| TEXAS INSTRUMENTS INCORPORATED
| Standard Linear and Logic Group
| IBIS Model of TS3DV416
| 4-CHANNEL DIFFERENTIAL 8:16 MULTIPLEXER SWITCH FOR DVI/HDMI
| APLICATIONS
| This file contains package information for the following:
|  TSSOP 48-pin (DGG) package as [Component] TS3DV416DB_DGG
|  TVSOP 48-pin (DGV) package as [Component] TS3DV416DB_DGV
| This device can be powered at the following Vccs:
|  3.3 volt Vcc
| This file provides unique models under the [Model Selector] for each Vcc.
| For operation at a specific Vcc, select the appropriate model after each
| [Model Selector] keyword.
[IBIS Ver]   3.2
[Comment char]  |_char
[File Name]   ts3dv416.ibs
[File Rev]   1.1 | b_die
[Date]   September 22, 2006
[Source]   Data created from TI-SPICE simulations at TI-SLL.
[Notes]   The following is an IBIS list for the TS3DV416.
   Please contact sllibis@ti.com with questions and
   comments concerning SLL IBIS models.
   - FILE REV HISTORY
   - 1.1 Release IBIS file on 09/22/06
   - Power clamp data deleted as there is no power-clamp diode.
[Disclaimer] Property of Texas Instruments Incorporated.  Unauthorized
   reproduction and/or distribution is strictly prohibited.
   This product is protected under copyright law.
   Created  2005, (C) Copyright  2005, Texas Instruments
   Incorporated, All Rights Reserved
   UNLESS THERE IS A SIGNED, WRITTEN AGREEMENT TO THE
   CONTRARY, TEXAS INSTRUMENTS (TI) IS PROVIDING THE IBIS
   MODELS  AND WITHOUT ANY WARRANTY, EXPRESSED OR
   IMPLIED.  TI assumes no liability for:
   1) the accuracy of the IBIS models provided to your
   company;
   2) the proper functioning of these IBIS Models in your
   design or for any resulting applications; or
   3) infringement of patents, copyrights or intellectual
   property rights resulting from your use of these IBIS
   models.
   TI provides IBIS Models as a service to our customers.
   You and your company shall not distribute, sell or give
   these models to anyone else without prior written
   permission from TI.
   TI reserves the right to make changes to our products or
   to discontinue any semiconductor product or service
   without notice, and advises our customers to obtain the
   latest version of relevant information to verify, before
   placing orders, that the information being relied on is
   current.
   Please be aware that your receipt and use of the IBIS
   information provided shall serve as acceptance of these
   terms and conditions.  If you do not accept these terms,
   you should return or destroy the IBIS models and any
   other accompanying information immediately.
| Component TS3DV416DB_DGG 48-pin TSSOP
[Component]   TS3DV416DB_DGG
[Manufacturer]   Texas Instruments, Inc.
[Package]
|   typ   min   max
R_pkg   6.200e-02   5.000e-02   7.800e-02
L_pkg   3.527e-09   3.128e-09   4.255e-09
C_pkg   5.300e-13   4.170e-13   6.850e-13
[Pin]   signal_name   model_name   R_pin   L_pin   C_pin
1   VDD   POWER   5.000e-02   4.250e-09   6.710e-13
2   A0   TS3DV416DB_A   5.700e-02   3.956e-09   6.740e-13
3   GND   GND   7.100e-02   3.922e-09   6.190e-13
4   A1   TS3DV416DB_A   7.800e-02   3.841e-09   6.180e-13
5   GND   GND   5.600e-02   3.535e-09   5.550e-13
6   VDD   POWER   5.800e-02   3.464e-09   5.030e-13
7   GND   GND   6.000e-02   3.362e-09   4.980e-13
8   A2   TS3DV416DB_A   6.100e-02   3.293e-09   4.620e-13
9   GND   GND   6.300e-02   3.240e-09   4.550e-13
10   A3   TS3DV416DB_A   6.300e-02   3.175e-09   4.420e-13
11   GND   GND   6.400e-02   3.153e-09   4.290e-13
12   VDD   POWER   6.500e-02   3.128e-09   4.180e-13
13   GND   GND   6.500e-02   3.128e-09   4.180e-13
14   NC   NC   6.400e-02   3.154e-09   4.290e-13
15   A4   TS3DV416DB_A   6.300e-02   3.174e-09   4.420e-13
16   GND   GND   6.300e-02   3.241e-09   4.550e-13
17   A5   TS3DV416DB_A   6.100e-02   3.293e-09   4.620e-13
18   GND   GND   6.000e-02   3.362e-09   4.970e-13
19   VDD   POWER   5.800e-02   3.464e-09   5.030e-13
20   GND   GND   5.600e-02   3.537e-09   5.600e-13
21   A6   TS3DV416DB_A   7.700e-02   3.839e-09   6.260e-13
22   GND   GND   7.100e-02   3.917e-09   6.270e-13
23   A7   TS3DV416DB_A   5.800e-02   3.955e-09   6.850e-13
24   SEL   TS3DV416DB_SEL   5.200e-02   4.255e-09   6.790e-13
25   7B2   TS3DV416DB_B2   5.100e-02   4.254e-09   6.760e-13
26   6B2   TS3DV416DB_B2   5.800e-02   3.957e-09   6.790e-13
27   GND   GND   7.100e-02   3.920e-09   6.210e-13
28   7B1   TS3DV416DB_B1   7.800e-02   3.843e-09   6.220e-13
29   6B1   TS3DV416DB_B1   5.600e-02   3.539e-09   5.600e-13
30   GND   GND   5.800e-02   3.466e-09   5.030e-13
31   5B2   TS3DV416DB_B2   6.000e-02   3.363e-09   4.970e-13
32   4B2   TS3DV416DB_B2   6.100e-02   3.294e-09   4.620e-13
33   GND   GND   6.300e-02   3.241e-09   4.540e-13
34   5B1   TS3DV416DB_B1   6.300e-02   3.175e-09   4.410e-13
35   4B1   TS3DV416DB_B1   6.400e-02   3.153e-09   4.290e-13
36   VDD   POWER   6.500e-02   3.129e-09   4.170e-13
37   GND   GND   6.500e-02   3.129e-09   4.170e-13
38   3B2   TS3DV416DB_B2   6.400e-02   3.152e-09   4.290e-13
39   2B2   TS3DV416DB_B2   6.400e-02   3.176e-09   4.410e-13
40   GND   GND   6.300e-02   3.241e-09   4.540e-13
41   3B1   TS3DV416DB_B1   6.100e-02   3.293e-09   4.620e-13
42   2B1   TS3DV416DB_B1   6.000e-02   3.363e-09   4.970e-13
43   GND   GND   5.800e-02   3.464e-09   5.030e-13
44   1B2   TS3DV416DB_B2   5.600e-02   3.534e-09   5.610e-13
45   0B2   TS3DV416DB_B2   7.800e-02   3.841e-09   6.260e-13
46   GND   GND   7.100e-02   3.920e-09   6.220e-13
47   1B1   TS3DV416DB_B1   5.700e-02   3.955e-09   6.770e-13
48   0B1   TS3DV416DB_B1   5.100e-02   4.252e-09   6.720e-13
| Component TS3DV416DB_DGV 48-pin TVSOP
[Component]   TS3DV416DB_DGV
[Manufacturer]   Texas Instruments, Inc.
[Package]
|   typ   min   max
R_pkg   7.000e-02   4.900e-02   8.500e-02
L_pkg   3.013e-09   2.743e-09   3.408e-09
C_pkg   3.710e-13   2.940e-13   5.110e-13
[Pin]   signal_name   model_name   R_pin   L_pin   C_pin
1   VDD   POWER   4.900e-02   3.393e-09   4.970e-13
2   A0   TS3DV416DB_A   6.000e-02   3.250e-09   5.020e-13
3   GND   GND   7.700e-02   3.310e-09   4.510e-13
4   A1   TS3DV416DB_A   8.500e-02   3.299e-09   4.040e-13
5   GND   GND   8.300e-02   3.136e-09   3.600e-13
6   VDD   POWER   7.700e-02   3.019e-09   3.630e-13
7   GND   GND   6.500e-02   2.882e-09   3.490e-13
8   A2   TS3DV416DB_A   6.600e-02   2.829e-09   3.140e-13
9   GND   GND   6.700e-02   2.796e-09   3.140e-13
10   A3   TS3DV416DB_A   6.900e-02   2.754e-09   3.080e-13
11   GND   GND   7.000e-02   2.753e-09   3.010e-13
12   VDD   POWER   7.100e-02   2.745e-09   2.940e-13
13   GND   GND   7.000e-02   2.744e-09   2.940e-13
14   NC   NC   7.000e-02   2.754e-09   3.010e-13
15   A4   TS3DV416DB_A   6.900e-02   2.754e-09   3.080e-13
16   GND   GND   6.700e-02   2.796e-09   3.140e-13
17   A5   TS3DV416DB_A   6.600e-02   2.829e-09   3.140e-13
18   GND   GND   6.500e-02   2.883e-09   3.500e-13
19   VDD   POWER   7.500e-02   3.014e-09   3.630e-13
20   GND   GND   8.000e-02   3.128e-09   3.580e-13
21   A6   TS3DV416DB_A   8.400e-02   3.295e-09   4.030e-13
22   GND   GND   7.800e-02   3.311e-09   4.520e-13
23   A7   TS3DV416DB_A   6.200e-02   3.259e-09   5.010e-13
24   SEL   TS3DV416DB_SEL   5.200e-02   3.404e-09   4.960e-13
25   7B2   TS3DV416DB_B2   5.300e-02   3.397e-09   5.050e-13
26   6B2   TS3DV416DB_B2   6.200e-02   3.249e-09   5.110e-13
27   GND   GND   7.700e-02   3.308e-09   4.530e-13
28   7B1   TS3DV416DB_B1   8.200e-02   3.289e-09   4.030e-13
29   6B1   TS3DV416DB_B1   7.800e-02   3.121e-09   3.590e-13
30   GND   GND   7.400e-02   3.010e-09   3.630e-13
31   5B2   TS3DV416DB_B2   6.500e-02   2.883e-09   3.490e-13
32   4B2   TS3DV416DB_B2   6.700e-02   2.829e-09   3.140e-13
33   GND   GND   6.700e-02   2.795e-09   3.140e-13
34   5B1   TS3DV416DB_B1   6.900e-02   2.753e-09   3.070e-13
35   4B1   TS3DV416DB_B1   7.000e-02   2.753e-09   3.010e-13
36   VDD   POWER   7.000e-02   2.743e-09   2.940e-13
37   GND   GND   7.000e-02   2.743e-09   2.940e-13
38   3B2   TS3DV416DB_B2   7.000e-02   2.753e-09   3.010e-13
39   2B2   TS3DV416DB_B2   6.900e-02   2.754e-09   3.070e-13
40   GND   GND   6.800e-02   2.797e-09   3.140e-13
41   3B1   TS3DV416DB_B1   6.700e-02   2.830e-09   3.140e-13
42   2B1   TS3DV416DB_B1   6.400e-02   2.880e-09   3.490e-13
43   GND   GND   7.200e-02   3.004e-09   3.620e-13
44   1B2   TS3DV416DB_B2   7.800e-02   3.121e-09   3.590e-13
45   0B2   TS3DV416DB_B2   8.400e-02   3.296e-09   4.030e-13
46   GND   GND   7.700e-02   3.308e-09   4.510e-13
47   1B1   TS3DV416DB_B1   6.200e-02   3.258e-09   4.990e-13
48   0B1   TS3DV416DB_B1   5.300e-02   3.408e-09   4.940e-13
[Series Switch Groups]
| Function Group States
On  1 /   | A1-A8->1B1-8B1 SEL LOW
   | 1B1-8B1->A1-A8 SEL LOW
On  2 /   | A1-A8->1B2-8B2 SEL HIGH
   | 1B2-8B2->A1-A8 SEL HIGH
[Series Pin Mapping]   pin_2   model_name   function_table_group
2   48   TS3DV416DB_A_S   1
4   47   TS3DV416DB_A_S   1
8   42   TS3DV416DB_A_S   1
10   41   TS3DV416DB_A_S   1
15   35   TS3DV416DB_A_S   1
17   34   TS3DV416DB_A_S   1
21   29   TS3DV416DB_A_S   1
23   28   TS3DV416DB_A_S   1
48   2   TS3DV416DB_B1_S   1
47   4   TS3DV416DB_B1_S   1
42   8   TS3DV416DB_B1_S   1
41   10   TS3DV416DB_B1_S   1
35   15   TS3DV416DB_B1_S   1
34   17   TS3DV416DB_B1_S   1
29   21   TS3DV416DB_B1_S   1
28   23   TS3DV416DB_B1_S   1
2   45   TS3DV416DB_A_S   2
4   44   TS3DV416DB_A_S   2
8   39   TS3DV416DB_A_S   2
10   38   TS3DV416DB_A_S   2
15   32   TS3DV416DB_A_S   2
17   31   TS3DV416DB_A_S   2
21   26   TS3DV416DB_A_S   2
23   25   TS3DV416DB_A_S   2
45   2   TS3DV416DB_B2_S   2
44   4   TS3DV416DB_B2_S   2
39   8   TS3DV416DB_B2_S   2
38   10   TS3DV416DB_B2_S   2
32   15   TS3DV416DB_B2_S   2
31   17   TS3DV416DB_B2_S   2
26   21   TS3DV416DB_B2_S   2
25   23   TS3DV416DB_B2_S   2
[Model]   TS3DV416DB_B1_S
Model_type  Series_switch
| variable   typ   min   max
C_comp   0   0   0
[Temperature Range]   40   100   -40
| Ambient temperature   25   85   -40
[Voltage range]   3.3   3   3.6
[On]
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[Off]
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[Model]   TS3DV416DB_B2_S
Model_type  Series_switch
| variable   typ   min   max
C_comp   0   0   0
[Temperature Range]   40   100   -40
| Ambient temperature   25   85   -40
[Voltage range]   3.3   3   3.6
[On]
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[Off]
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[Model]   TS3DV416DB_A_S
Model_type  Series_switch
| variable   typ   min   max
C_comp   0   0   0
[Temperature Range]   40   100   -40
| Ambient temperature   25   85   -40
[Voltage range]   3.3   3   3.6
[On]
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[Off]
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| Models and submodels in the file (7): TS3DV416DB_SEL (Input), TS3DV416DB_B1_S (Series_switch), TS3DV416DB_B1 (Terminator), TS3DV416DB_B2_S (Series_switch), TS3DV416DB_B2 (Terminator), TS3DV416DB_A_S (Series_switch), TS3DV416DB_A (Terminator)
